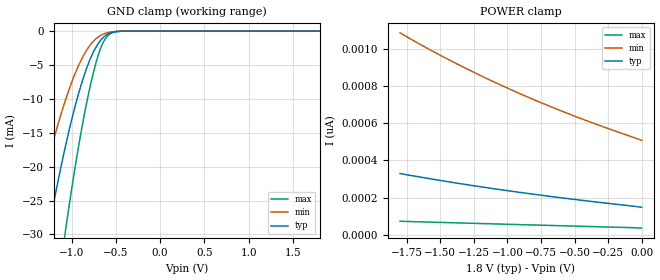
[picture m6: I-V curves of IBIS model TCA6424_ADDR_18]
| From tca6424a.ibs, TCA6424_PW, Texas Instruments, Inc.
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[Model]   TCA6424_ADDR_18
Model_type  Input
Vinl=0.495
Vinh=1.365
| variable   typ   min   max
C_comp   2.22pF   1.67pF   2.46pF
[Temperature Range]   40   100   -40
| Ambient temperature   25   85   -40
[Voltage range]   1.8   1.65   1.95
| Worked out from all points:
|   GND clamp passes 1 mA (typ) near -0.65 V on its own axis
[GND Clamp]
| TCA6424_ADDR_18
|   Voltage   I(typ)   I(min)   I(max)
-1.8V     -74.02mA   -51.67mA   -111.7mA
-1.45V    -43.77mA   -29.21mA   -69.33mA
-1.27V    -30.12mA   -19.36mA   -49.42mA
-1.25V    -28.7mA    -18.35mA   -47.31mA
-1.07V    -17.07mA   -10.25mA   -29.6mA
-960mV    -11.11mA   -6.281mA   -20.1mA
-855mV    -6.438mA   -3.375mA   -12.27mA
-765mV    -3.406mA   -1.667mA   -6.757mA
-680mV    -1.498mA   -708.4uA   -2.836mA
-590mV    -450.5uA   -228.8uA   -677.8uA
-475mV    -54.97uA   -37.86uA   -56.06uA
1.8V      147.6pA    546pA      30.99pA
[POWER Clamp]
| TCA6424_ADDR_18
|   Voltage   I(typ)   I(min)   I(max)
-1.8V     329.2pA    1.086nA    72.27pA
-1.605V   304.6pA    1.007nA    68.21pA
-1.385V   278.5pA    922.7pA    63.7pA
-1.17V    254.7pA    846.2pA    59.35pA
-950mV    231.9pA    773pA      54.95pA
-730mV    210.6pA    704.8pA    50.6pA
-505mV    190.2pA    639.7pA    46.2pA
-290mV    171.9pA    581.8pA    42.03pA
-16.28fV  147.6pA    508.2pA    35.04pA
